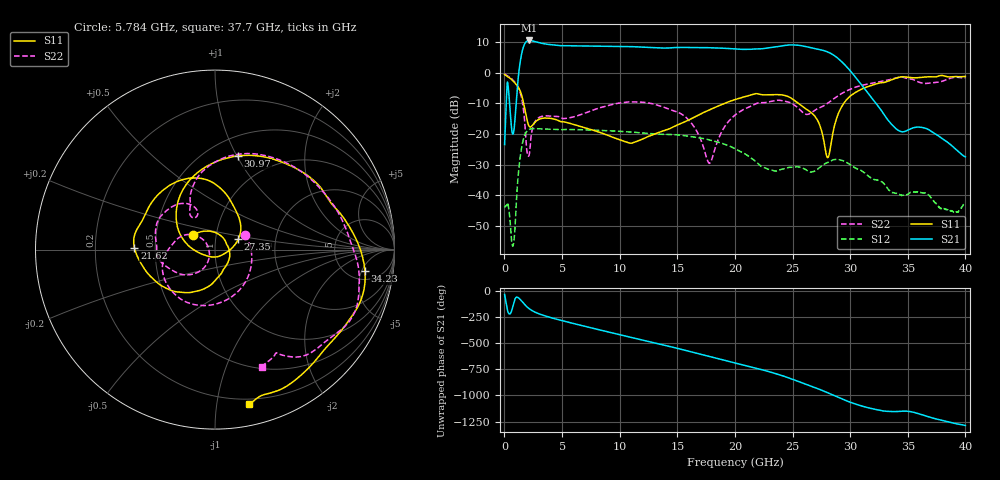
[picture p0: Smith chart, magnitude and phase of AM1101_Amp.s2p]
!Agilent Technologies,E8364B,MY43040894,A.07.50.67
!Agilent E8364B: A.07.50.67
!Date: Tuesday, June 02, 2020 10:43:55
!Correction: S11(Full 2 Port(1,2))
!S21(Full 2 Port(1,2))
!S12(Full 2 Port(1,2))
!S22(Full 2 Port(1,2))
!S2P File: Measurements: S11, S21, S12, S22:
# Hz S  dB  R 50
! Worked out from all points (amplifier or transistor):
!   6401 points, 10 MHz to 40 GHz, reference 50 ohm
!   highest |S21| = 10.5 dB at 2.159 GHz (marker M1)
!   |S21| within 3 dB of that: 1.571 GHz to 27.39 GHz (25.81 GHz wide, 178 % of centre)
!   unconditionally stable (mu >= 1): start of sweep to end of sweep
!   at 6.671 GHz: K = 1.65, MAG = 8.9 dB, |S12| = -18.6 dB
!   at 20 GHz: K = 3.08, MAG = 8.5 dB, |S12| = -24.7 dB
!   at 40 GHz: K = 119.57, MAG = -16.3 dB, |S12| = -42.3 dB
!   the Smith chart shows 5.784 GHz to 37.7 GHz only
!   S11 on the Smith chart (normalised r, x): 5.784 GHz: 0.77, +0.13; 21.62 GHz: 0.38, +0.01; 27.35 GHz: 1.29, +0.15; 30.97 GHz: 0.69, +1.01; 34.23 GHz: 6.97, -5.76; 37.7 GHz: 0.16, -1.23
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1e7  -0.59 -13.3  -23.42 -36.2  -43.88 32.3  -0.41 -12.8
1.297178e9  -5.42 148.6  1.77 -75.5  -29.46 153.6  -5.73 154.9
1.697078e9  -10.63 73.6  8.96 -124.7  -20.95 97.9  -13.67 96.8
2.159462e9  -17.53 -38.9  10.51 -173.0  -18.46 44.8  -26.45 177.9
3.515373e9  -14.77 -164.9  9.38 119.9  -18.36 -30.5  -14.07 131.4
5.783556e9  -16.62 146.4  8.77 52.6  -18.51 -102.8  -14.57 25.8
6.677083e9  -17.57 133.2  8.70 28.2  -18.58 -127.8  -13.60 -11.2
1.04199e10  -22.39 44.4  8.51 -70.8  -19.17 133.2  -9.64 -113.3
1.334417e10  -19.53 -50.8  8.06 -147.8  -20.00 59.2  -10.64 -168.4
1.523119e10  -16.67 -80.1  8.26 163.5  -20.35 9.6  -13.20 164.3
1.723069e10  -13.05 -104.2  8.18 108.4  -21.41 -45.7  -23.81 142.7
2.0005e10  -8.76 -148.0  7.75 30.0  -24.75 -125.1  -13.83 -136.3
2.16171e10  -6.96 178.8  7.71 -13.9  -28.37 -166.3  -10.47 -164.2
2.439765e10  -7.48 109.8  8.93 -101.9  -31.13 160.7  -9.33 137.6
2.667208e10  -13.19 51.9  8.06 165.7  -32.36 107.4  -12.90 125.8
2.734691e10  -16.97 23.9  7.54 137.8  -30.89 100.1  -11.44 121.3
2.914646e10  -11.87 146.4  4.02 52.4  -28.46 32.1  -7.03 98.3
3.097101e10  -5.38 76.2  -3.84 -20.1  -31.88 -29.9  -4.18 53.3
3.333917e10  -2.67 14.5  -15.68 -72.7  -38.18 -81.9  -2.35 1.7
3.423269e10  -1.48 -8.1  -18.91 -72.8  -39.68 -83.9  -1.47 -19.1
3.770058e10  -1.07 -77.7  -20.70 -151.7  -43.84 -142.4  -3.06 -68.4
4e10  -1.22 -114.5  -27.44 153.1  -42.35 -140.3  -1.64 -105.9
